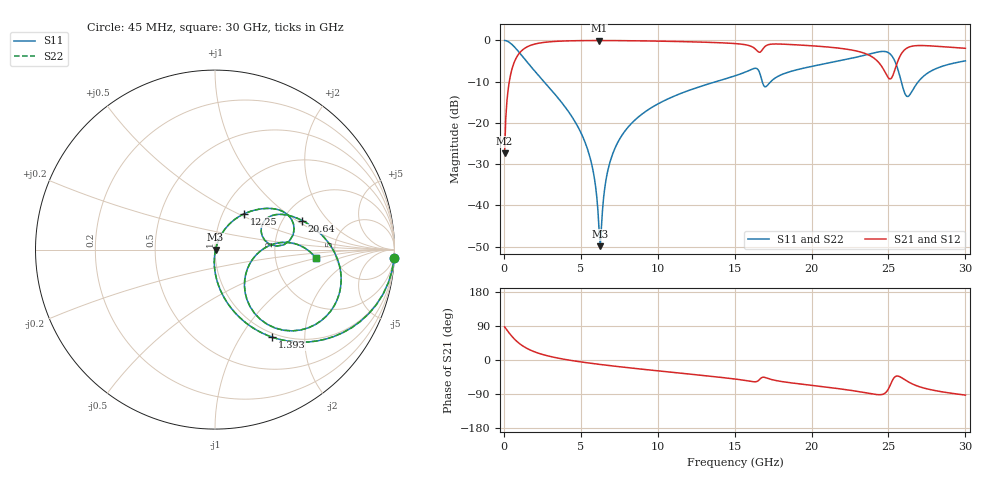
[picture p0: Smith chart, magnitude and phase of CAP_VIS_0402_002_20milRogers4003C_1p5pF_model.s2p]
! S-parameter model data by Modelithics Inc.  support@modelithics.com  813-866-6335  Tampa FL USA
! S-Parameter data specifications:
! Substrate: 20-mil Rogers 4003C, substrate thickness, H=0.508mm, Dielectric constant, Er=3.75
! PCB Mounting Pad Footprint: Pad width, PadW=0.50mm , Pad length, PadL=0.50mm , Pad gap, PadG (edge-to-edge)=0.40mm , Reference planes=1.4mm apart
! Created Wed Nov 18 12:34:22 2015
# hz S ma R 50
! 2 Port Network Data from SP1.SP block
! freq  magS11  angS11  magS21  angS21  magS12  angS12  magS22  angS22
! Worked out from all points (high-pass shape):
!   401 points, 45 MHz to 30 GHz, reference 50 ohm
!   highest |S21| = -0.03 dB at 6.186 GHz (marker M1); lowest = -27.3 dB at 45 MHz (marker M2)
!   |S21| within 3 dB of the highest: 1.018 GHz to 23.37 GHz (22.36 GHz wide, 183 % of centre); 25.88 GHz to end of sweep
!   lowest |S11| = -49.9 dB at 6.261 GHz (marker M3), VSWR 1.01, Z = 50.3 - j0.0506 ohm
!   |S11| at or under -10 dB: 2.604 GHz to 13.78 GHz (11.18 GHz wide, 136 % of centre); 16.79 GHz to 17.35 GHz (551.6 MHz wide, 3.23 % of centre); 25.83 GHz to 26.94 GHz (1.108 GHz wide, 4.2 % of centre)
!   |S22| runs from -49.9 to 0.0 dB; largest |S21 - S12| = 0
!   S11 on the Smith chart (normalised r, x): 45 MHz: 1, -45; 1.393 GHz: 0.94, -1.38; 12.25 GHz: 1.26, +0.54; 20.64 GHz: 2.54, +1.11; 30 GHz: 3.52, -0.49
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4.5e7  0.9991 -2.5  0.04291 87.5  0.04291 87.5  0.9991 -2.5
4.94325e8  0.9032 -26.3  0.4288 63.7  0.4288 63.7  0.9032 -26.3
1.392975e9  0.5814 -57.0  0.8123 32.9  0.8123 32.9  0.5814 -57.0
2.666062e9  0.3068 -76.8  0.9497 12.8  0.9497 12.8  0.3068 -76.8
5.062462e9  0.07222 -93.1  0.9944 -5.4  0.9944 -5.4  0.07222 -93.1
5.73645e9  0.02977 -93.2  0.9963 -9.1  0.9963 -9.1  0.02977 -93.2
6.185775e9  0.005068 -62.6  0.9966 -11.4  0.9966 -11.4  0.005068 -62.6
6.260662e9  0.003201 -9.0  0.9966 -11.8  0.9966 -11.8  0.003201 -9.0
6.709988e9  0.02413 68.1  0.9962 -14.0  0.9962 -14.0  0.02413 68.1
7.309088e9  0.05366 69.4  0.9949 -16.8  0.9949 -16.8  0.05366 69.4
1.007992e10  0.1726 59.7  0.9804 -28.9  0.9804 -28.9  0.1726 59.7
1.225166e10  0.2564 50.9  0.961 -37.9  0.961 -37.9  0.2564 50.9
1.50225e10  0.3723 38.0  0.9162 -50.2  0.9162 -50.2  0.3723 38.0
1.674491e10  0.3409 3.3  0.7458 -46.8  0.7458 -46.8  0.3409 3.3
2.003996e10  0.4856 21.4  0.8605 -67.1  0.8605 -67.1  0.4856 21.4
2.063906e10  0.5117 18.5  0.8445 -70.0  0.8445 -70.0  0.5117 18.5
2.348479e10  0.6638 -1.0  0.6938 -86.3  0.6938 -86.3  0.6638 -1.0
2.505742e10  0.6978 -36.8  0.3424 -71.2  0.3424 -71.2  0.6978 -36.8
2.573141e10  0.3725 -58.4  0.634 -44.0  0.634 -44.0  0.3725 -58.4
2.625562e10  0.2087 -23.7  0.818 -57.0  0.818 -57.0  0.2087 -23.7
2.767849e10  0.4164 5.4  0.8597 -77.8  0.8597 -77.8  0.4164 5.4
3e10  0.5651 -4.8  0.8024 -92.6  0.8024 -92.6  0.5651 -4.8
